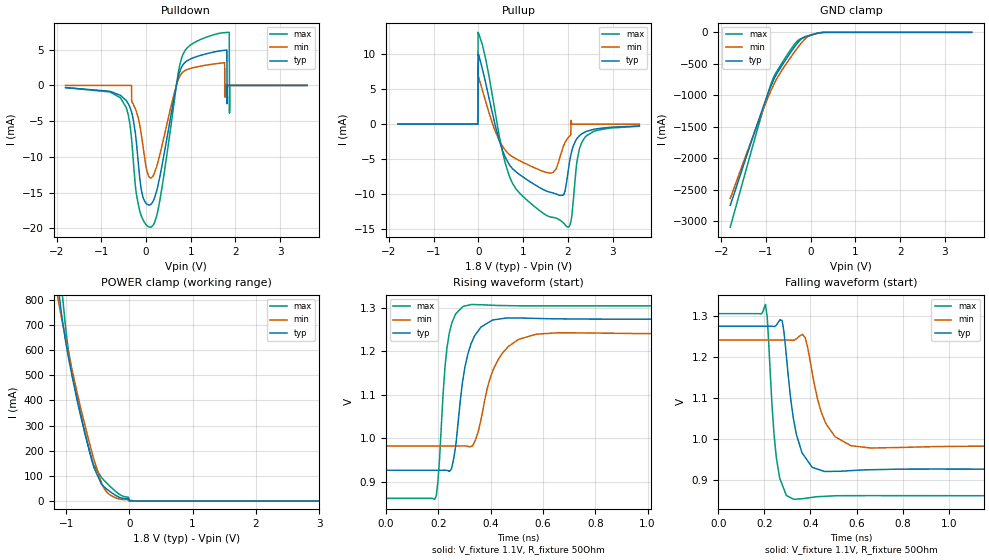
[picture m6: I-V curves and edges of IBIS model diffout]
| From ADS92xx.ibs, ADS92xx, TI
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|   diffout Model
[Model]   diffout
Model_type   3-state
Polarity   Non-Inverting
Vmeas = 0.9
Vref = 0.9
Cref = 2pF
Rref = 50
|   typ   min   max
C_comp   2.8pF   2.47pF   3.46pF
[Voltage Range]   1.8   1.75   1.85
[Temperature Range]   27   125   -40
[Pullup Reference]   1.8   1.75   1.85
[Pulldown Reference]   0   0   0
[Power Clamp Reference]   1.8   1.75   1.85
[GND Clamp Reference]   0   0   0
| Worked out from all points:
|   slope of the pulldown table from 0 to 0.27 V, typ, clamps not added: 103 ohm
|   slope of the pullup table from 0 to 0.27 V, typ, clamps not added: 37.7 ohm
|   falling waveform, V_fixture 1.1V, R_fixture 50Ohm: 20-80 % time 52ps typ, 71.8ps min, 32.6ps max; typ from 1.27 V to 0.926 V
|   rising waveform, V_fixture 1.1V, R_fixture 50Ohm: 20-80 % time 49.3ps typ, 77.8ps min, 30.7ps max; typ from 0.926 V to 1.27 V
[Pulldown]
|   Voltage   I(typ)   I(min)   I(max)
-1.8V     -311.2uA   0A         -312.2uA
-574.2mV  -1.395mA   0A         -1.737mA
-325.8mV  -3.719mA   0A         -7.423mA
-169.2mV  -11.17mA   -4.721mA   -16.79mA
84.6mV    -16.73mA   -12.94mA   -19.85mA
916.2mV   3.439mA    2.218mA    5.235mA
1.807V    4.951mA    15.9pA     7.405mA
1.813V    -2.569mA   -4.7pA     7.407mA
1.861V    -11.75nA   -30.2pA    7.428mA
1.867V    11.67nA    -30.2pA    -3.881mA
1.872V    -11.57nA   -30.2pA    -103.8nA
3.6V      21nA       0A         5.7nA
[GND Clamp]
|   Voltage   I(typ)   I(min)   I(max)
-1.8V     -2.75A     -2.64A     -3.097A
-1.195V   -1.458A    -1.466A    -1.549A
-1.006V   -1.072A    -1.122A    -1.084A
-887.4mV  -850mA     -924.6mA   -816.2mA
-790.2mV  -697.1mA   -777.8mA   -657.9mA
-639mV    -521mA     -596.4mA   -482.6mA
-444.6mV  -313mA     -393.8mA   -269.7mA
-288mV    -162.9mA   -239.1mA   -131.1mA
-180mV    -89.31mA   -145.1mA   -89.8mA
-61.2mV   -54.35mA   -67.19mA   -63.37mA
246.6mV   -3.307mA   -4.267mA   -2.242mA
3.6V      0A         0A         0A
[Pullup]
|   Voltage   I(typ)   I(min)   I(max)
-1.8V     0A         0A         0A
-18mV     -12.41nA   300fA      0A
-12.6mV   9.375nA    200fA      1.843mA
-7.2mV    3.157nA    200fA      13.08mA
-1.8mV    10mA       6.798mA    13mA
721.8mV   -6.038mA   -4.474mA   -7.863mA
1.651V    -9.775mA   -6.933mA   -13.27mA
1.904V    -10.07mA   -3.096mA   -14.09mA
2.018V    -6.241mA   -1.849mA   -14.68mA
2.218V    -1.94mA    10pA       -4.828mA
2.38V     -1.138mA   10pA       -1.915mA
3.6V      -258.2uA   0A         -300.2uA
[POWER Clamp]
|   Voltage   I(typ)   I(min)   I(max)
-1.8V     2.754A     2.329A     3.187A
-1.179V   981.3mA    878.7mA    1.164A
-1.109V   816.2mA    774.9mA    953.9mA
-1.071V   739.1mA    724.7mA    847.2mA
-1.001V   622.2mA    636.2mA    671.8mA
-898.2mV  485.9mA    512.8mA    498.1mA
-595.8mV  162.9mA    196.5mA    167.6mA
-428.4mV  64.08mA    65.54mA    90.33mA
-282.6mV  33.7mA     21.02mA    53.31mA
-7.2mV    8.839mA    5.354mA    3.641mA
117mV     239.6uA    78.43uA    939.5uA
3.6V      0A         0A         0A
[Ramp]
R_load = 50
|   typ   min   max
dV/dt_r   0.209084/4.93349e-11   0.155278/7.77697e-11   0.266373/3.06623e-11
dV/dt_f   0.209051/5.20253e-11   0.15526/7.17497e-11   0.266254/3.26058e-11
[Falling Waveform]
V_fixture = 1.1V
V_fixture_min = 1.1V
V_fixture_max = 1.1V
R_fixture = 50Ohm
C_fixture = 0F
|   Time   V(typ)   V(min)   V(max)
0s        1.275V     1.241V     1.305V
205.3ps   1.275V     1.241V     1.328V
252.1ps   1.277V     1.241V     954.3mV
277.5ps   1.288V     1.241V     888.5mV
327.8ps   1.044V     1.241V     852.7mV
377.5ps   954.8mV    1.247V     855.2mV
407.9ps   930.5mV    1.161V     857.7mV
467.9ps   920.6mV    1.036V     860.2mV
575.7ps   922.7mV    983.4mV    861.6mV
1.673ns   926.3mV    982.2mV    861.6mV
[Rising Waveform]
V_fixture = 1.1V
V_fixture_min = 1.1V
V_fixture_max = 1.1V
R_fixture = 50Ohm
C_fixture = 0F
|   Time   V(typ)   V(min)   V(max)
0s        926.1mV    982.1mV    861.3mV
192.5ps   926.1mV    982.1mV    866.5mV
233.6ps   925.7mV    982.1mV    1.208V
259.6ps   953.9mV    982.1mV    1.277V
295.6ps   1.139V     982.2mV    1.304V
330.8ps   1.225V     981.8mV    1.308V
363.4ps   1.256V     1.043V     1.308V
412.2ps   1.273V     1.161V     1.306V
507.4ps   1.277V     1.228V     1.305V
1.673ns   1.275V     1.241V     1.305V
